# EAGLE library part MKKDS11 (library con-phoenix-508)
PHOENIX
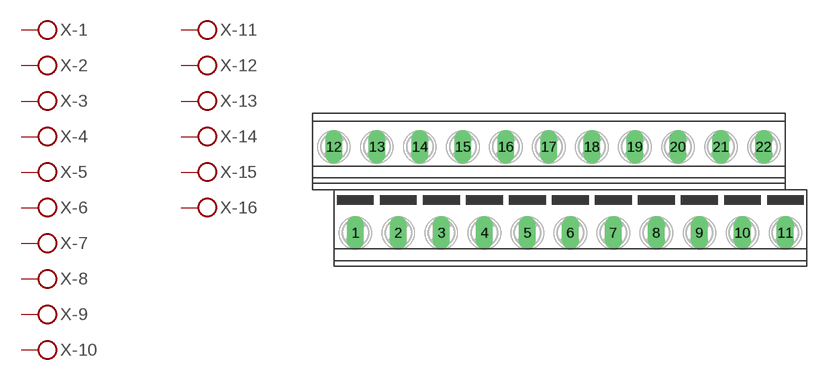
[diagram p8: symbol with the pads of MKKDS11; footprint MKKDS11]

Designator prefix X; gates -1=KL -2=KL -3=KL -4=KL -5=KL -6=KL -7=KL -8=KL -9=KL -10=KL -11=KL -12=KL -13=KL -14=KL -15=KL -16=KL -17=KL -18=KL -19=KL -20=KL -21=KL -22=KLV

## MKKDS11 (OC_FARNELL: unknown; OC_NEWARK: unknown)  [MKKDS11]
1  -1:KL  pas
2  -2:KL  pas
3  -3:KL  pas
4  -4:KL  pas
5  -5:KL  pas
6  -6:KL  pas
7  -7:KL  pas
8  -8:KL  pas
9  -9:KL  pas
10  -10:KL  pas
11  -11:KL  pas
12  -12:KL  pas
13  -13:KL  pas
14  -14:KL  pas
15  -15:KL  pas
16  -16:KL  pas
17  -17:KL  pas
18  -18:KL  pas
19  -19:KL  pas
20  -20:KL  pas
21  -21:KL  pas
22  -22:KL  pas

## Footprint MKKDS11 (pad centres in mm)
PHOENIX MKKDSN 1,5/ 8-5,08 Source: http://eshop.phoenixcontact.com .. 1726202.pdf
drill 1.321 long: 1 -24.13,-5.08; 2 -19.05,-5.08; 3 -13.97,-5.08; 4 -8.89,-5.08; 5 -3.81,-5.08; 6 1.27,-5.08; 7 6.35,-5.08; 8 11.43,-5.08; 9 16.51,-5.08; 10 21.59,-5.08; 11 26.67,-5.08; 12 -26.67,5.08; 13 -21.59,5.08; 14 -16.51,5.08; 15 -11.43,5.08; 16 -6.35,5.08; 17 -1.27,5.08; 18 3.81,5.08; 19 8.89,5.08; 20 13.97,5.08; 21 19.05,5.08; 22 24.13,5.08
